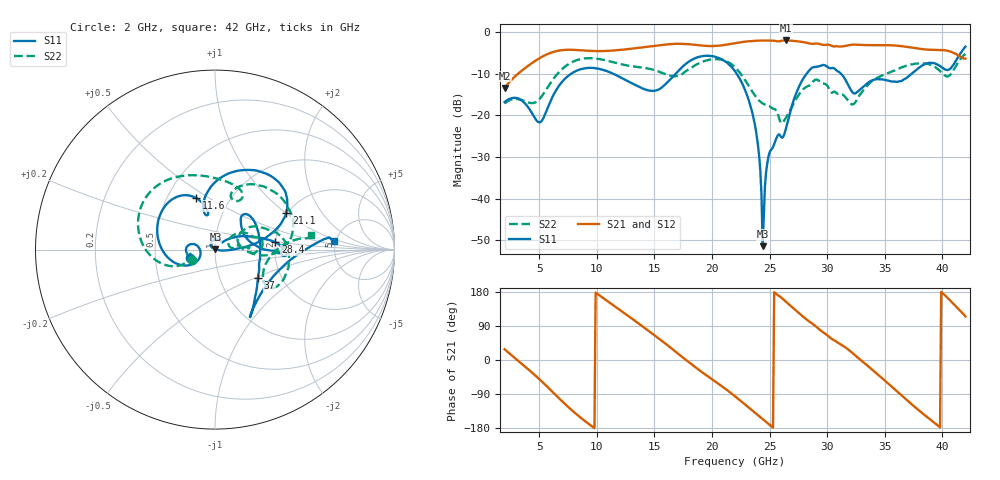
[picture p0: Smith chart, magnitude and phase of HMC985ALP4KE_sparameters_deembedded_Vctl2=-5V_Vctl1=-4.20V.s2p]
!s2p File: Measurements: S11, S21, S12, S22
# GHz S dB R 50.0
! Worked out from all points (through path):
!   401 points, 2 GHz to 42 GHz, reference 50 ohm
!   highest |S21| = -2.07 dB at 26.4 GHz (marker M1); lowest = -13.4 dB at 2 GHz (marker M2)
!   lowest |S11| = -51.4 dB at 24.4 GHz (marker M3), VSWR 1.01, Z = 50.3 + j0.0841 ohm
!   |S11| at or under -10 dB: start of sweep to 7.806 GHz; 22.14 GHz to 28.23 GHz (6.091 GHz wide, 24.2 % of centre); 31.18 GHz to 37.36 GHz (6.18 GHz wide, 18 % of centre)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
!   |S22| runs from -21.9 to -5.3 dB; largest |S21 - S12| = 0.00094
!   S11 on the Smith chart (normalised r, x): 2 GHz: 0.76, -0.07; 11.6 GHz: 0.69, +0.44; 21.1 GHz: 1.97, +1.01; 28.4 GHz: 2.00, +0.19; 37 GHz: 1.52, -0.53; 42 GHz: 4.81, +0.81
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2  -16.84 -161.9  -13.44 28.2  -13.45 28.2  -17.16 -155.8
5  -21.72 -172.9  -6.39 -50.1  -6.39 -50.1  -16.20 -160.0
6.3  -14.84 -150.7  -4.77 -88.3  -4.77 -88.3  -11.05 -161.6
8.7  -8.90 150.2  -4.45 -154.6  -4.45 -154.6  -6.48 151.3
11.6  -10.28 110.2  -4.45 140.9  -4.45 140.9  -7.41 103.5
13.6  -13.11 101.0  -3.85 97.1  -3.85 97.1  -8.46 75.9
15.4  -13.80 105.7  -3.25 56.3  -3.25 56.3  -9.54 62.5
17.9  -7.32 80.0  -2.95 -3.7  -2.95 -3.7  -9.14 72.3
21.1  -7.00 27.3  -3.14 -74.6  -3.14 -74.5  -6.88 16.0
22  -9.43 16.7  -2.71 -95.8  -2.71 -95.7  -8.49 0.6
23.6  -20.57 -0.2  -2.18 -135.5  -2.18 -135.5  -14.76 -3.7
24  -27.33 -7.1  -2.11 -145.6  -2.12 -145.5  -16.22 1.9
24.4  -51.41 18.1  -2.09 -155.7  -2.09 -155.6  -17.17 7.6
25  -28.92 133.2  -2.12 -170.9  -2.12 -170.9  -17.85 11.1
26.4  -23.43 43.2  -2.07 154.3  -2.07 154.4  -20.71 33.0
28.4  -9.40 7.1  -2.75 102.4  -2.75 102.4  -12.95 18.3
28.7  -8.60 2.0  -2.88 96.2  -2.88 96.2  -12.21 16.5
32.5  -14.65 33.7  -3.09 10.4  -3.08 10.4  -16.64 29.0
35.4  -11.76 18.8  -3.21 -65.0  -3.21 -65.0  -9.79 19.4
37  -10.82 -33.6  -3.63 -108.1  -3.63 -108.0  -8.02 5.0
39.8  -8.21 -56.7  -4.34 -177.6  -4.34 -177.6  -9.40 -34.8
42  -3.56 4.1  -6.42 114.9  -6.42 114.9  -5.30 8.7
